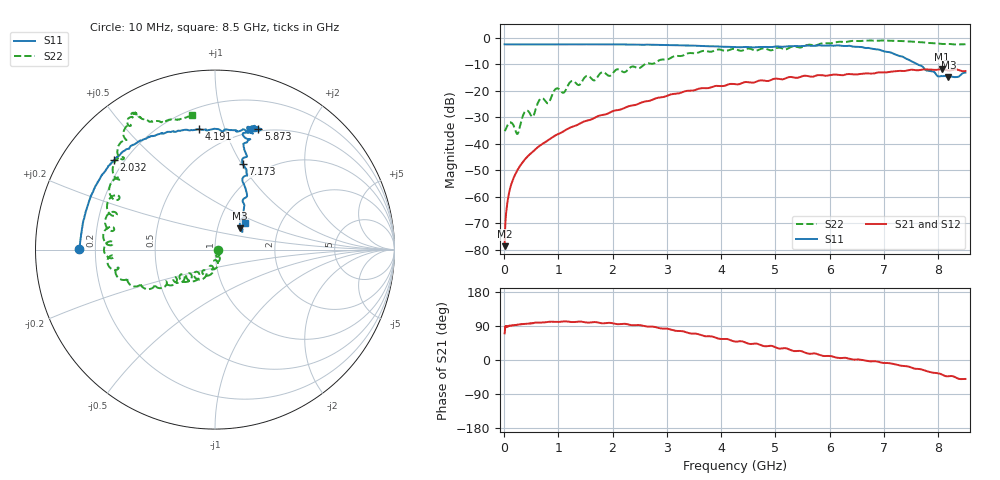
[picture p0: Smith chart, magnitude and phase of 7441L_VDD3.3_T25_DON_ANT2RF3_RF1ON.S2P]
!Agilent Technologies,E5071C,MY46417908,A.11.23
!Date: Mon May 03 19:53:42 2021
!Data & Calibration Information:
!Freq	S11:SOLT2(ON)	S21:SOLT2(ON)	S12:SOLT2(ON)	S22:SOLT2(ON)
!PortZ  Port1:50+j0  Port2:50+j0
!Above PortZ is port z conversion or system Z0 setting when saving the data.
!When reading, reference impedance value at option line is always used.
# Hz S dB R 50
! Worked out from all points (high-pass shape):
!   1601 points, 10 MHz to 8.5 GHz, reference 50 ohm
!   highest |S21| = -11.76 dB at 8.065 GHz (marker M1); lowest = -78.6 dB at 10 MHz (marker M2)
!   |S21| within 3 dB of the highest: 5.27229 GHz to 5.293522 GHz (21.23 MHz wide, 0.402 % of centre); 5.457 GHz to end of sweep
!   lowest |S11| = -14.9 dB at 8.187 GHz (marker M3), VSWR 1.44, Z = 63.7 + j15.5 ohm
!   |S11| at or under -10 dB: 7.619 GHz to end of sweep
!   |S22| runs from -36.3 to -1.0 dB; largest |S21 - S12| = 0.002
!   S11 on the Smith chart (normalised r, x): 10 MHz: 0.14, +0.00; 2.032 GHz: 0.16, +0.37; 4.191 GHz: 0.33, +0.82; 5.873 GHz: 0.48, +1.31; 7.173 GHz: 0.79, +1.01; 8.5 GHz: 1.32, +0.41
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1e7  -2.42 179.7  -78.57 70.5  -77.39 75.1  -35.16 -0.7
6.30625e7  -2.47 178.5  -61.79 87.5  -61.70 89.6  -33.04 -12.1
1.108188e8  -2.47 177.2  -56.75 90.4  -56.68 90.2  -31.94 -32.3
2.43475e8  -2.49 174.4  -50.00 93.3  -49.99 93.1  -36.21 -49.4
3.230688e8  -2.50 172.5  -47.46 94.7  -47.41 94.7  -30.92 -36.8
4.079688e8  -2.51 170.5  -45.33 95.5  -45.34 95.5  -27.46 -64.4
5.353188e8  -2.49 167.8  -42.84 97.4  -42.84 97.3  -29.61 -67.7
6.732812e8  -2.50 164.6  -40.45 98.8  -40.47 98.7  -22.95 -77.0
8.218562e8  -2.50 161.4  -38.47 100.6  -38.47 100.7  -24.50 -84.4
9.545125e8  -2.48 158.4  -36.69 100.6  -36.72 100.6  -19.22 -92.1
1.426769e9  -2.46 149.5  -31.98 101.2  -31.99 101.1  -16.79 -109.1
2.031681e9  -2.48 138.6  -27.45 96.0  -27.46 96.0  -12.59 -130.4
2.843538e9  -2.64 125.6  -22.56 84.7  -22.57 84.7  -8.64 -144.5
4.191325e9  -3.39 97.6  -17.36 51.2  -17.37 51.2  -4.26 -177.6
4.255e9  -3.47 94.8  -17.46 48.7  -17.46 48.7  -4.23 177.9
5.671769e9  -3.01 69.5  -14.67 16.7  -14.62 16.5  -2.69 135.4
5.873406e9  -2.95 70.2  -14.13 10.9  -14.07 11.1  -2.01 132.1
7.088538e9  -5.37 72.3  -12.87 -8.4  -12.90 -8.3  -1.09 120.4
7.173438e9  -5.98 72.1  -12.65 -10.4  -12.66 -10.3  -1.11 120.4
8.064888e9  -14.43 36.0  -11.76 -38.2  -11.77 -38.2  -2.29 112.3
8.186931e9  -14.86 40.7  -12.36 -42.9  -12.41 -42.7  -2.30 109.4
8.5e9  -13.12 41.8  -12.54 -50.0  -12.59 -50.0  -2.41 99.6
